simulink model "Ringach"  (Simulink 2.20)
settings: Solver=ode45  StartTime=0.0  StopTime=3  RelTol=1e-3  AbsTol=1e-6
libraries: simulink x1

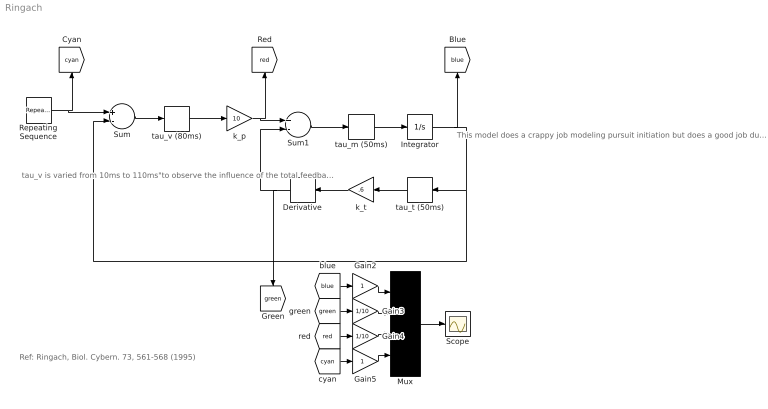
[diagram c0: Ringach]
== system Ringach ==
  note: tau_v is varied from 10ms to 110ms"to observe the influence of the total feedback delay tau_tot=tau_v+tau_m."
  note: Ref: Ringach, Biol. Cybern. 73, 561-568 (1995)
  note: This model does a crappy job modeling pursuit initiation but does a good job during steady state. It uses an accelleration signal but computes it off eye velocity not off the forward pathway . That's why it blows onset this is the property that steve is planning to exploit.
  Derivative : Derivative  Orientation=left
  Gain2 : Gain  Gain=1
  Gain3 : Gain  Gain=1/10
  Gain4 : Gain  Gain=1/10
  Gain5 : Gain  Gain=1
  Integrator : Integrator  ExternalReset=none  InitialConditionSource=internal  InitialCondition=0  LimitOutput=off  UpperSaturationLimit=inf  LowerSaturationLimit=-inf  ShowSaturationPort=off  ShowStatePort=off  AbsoluteTolerance=auto
  Mux : Mux  Inputs=4
  Repeating Sequence : simulink/Sources/Repeating Sequence  rep_seq_t=[0 .1 .10001 3 3.0001 6]  rep_seq_y=[0 0 20 20 0 0]
  Scope : Scope
  Sum : Sum  Inputs=+-
  Sum1 : Sum  Inputs=+-
  k_p : Gain  Gain=10
  k_t : Gain  Orientation=left  Gain=.6
  tau_m (50ms) : TransportDelay  DelayTime=50e-3  InitialInput=0  BufferSize=1024
  tau_t (50ms) : TransportDelay  Orientation=left  DelayTime=50e-3  InitialInput=0  BufferSize=1024
  tau_v (80ms) : TransportDelay  DelayTime=80e-3  InitialInput=0  BufferSize=1024
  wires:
  tau_t (50ms)/1 -> k_t/1
  k_t/1 -> Derivative/1
  tau_v (80ms)/1 -> k_p/1
  Sum1/1 -> tau_m (50ms)/1
  tau_m (50ms)/1 -> Integrator/1
  Sum/1 -> tau_v (80ms)/1
  Repeating Sequence/1 -> Sum/1, [cyan]
  k_p/1 -> Sum1/1, [red]
  Integrator/1 -> tau_t (50ms)/1, Sum/2, [blue]
  Derivative/1 -> Sum1/2, [green]
  Mux/1 -> Scope/1
  [blue] -> Gain2/1
  Gain2/1 -> Mux/1
  [green] -> Gain3/1
  Gain3/1 -> Mux/2
  [red] -> Gain4/1
  Gain4/1 -> Mux/3
  [cyan] -> Gain5/1
  Gain5/1 -> Mux/4
